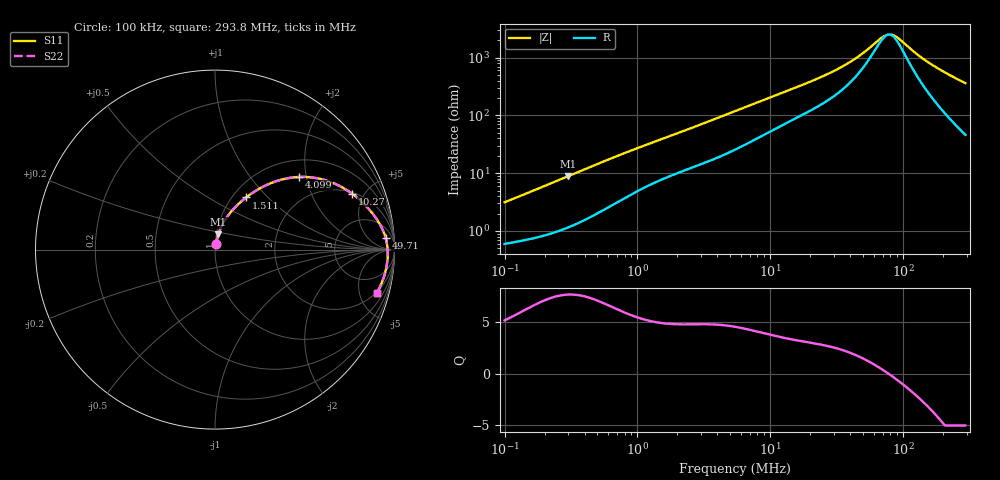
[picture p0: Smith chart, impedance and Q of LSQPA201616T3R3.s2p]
! LSQPA201616T3R3  S-PARAMETER MODEL  ( General Type )
! Model Generated by TAIYO YUDEN Corporation (http://www.ty-top.com)
! Version 2.0
! TAIYO YUDEN Control No. 100810NF25SB-FKC
! Copyright(c) 2007 TAIYO YUDEN CO.,LTD. All Rights Reserved.
! Product Description (link to TY-COMPAS)
! https://ds.yuden.co.jp/TYCOMPAS/or/detail?pn=LSQPA201616T3R3M&u=M
! Products Name : Inductors
! Characteristics :
!  Inductance : 3.3 uH , SRF(min) : 55 MHz , DC Resistance(max) : 0.351 Ohm
!  Rated Current : Saturation :600 mA , Temp Rise : 610 mA (40 degC)
!  Case Size : 2.0 x 1.6 / 0.079 x 0.063 [mm/inch] , Thickness : 1.6 / 0.063 [mm/inch]
!  (Conditions: Temperature = 25 degC , DC Bias Current/Voltage = 0A / 0V)
! External Node Assignments :
!  1  o---GGG---o  2
! GND o---------o GND
! Frequency Range : 0.1MHz  -  293.796821MHz  [ 402 STEP ]
# MHz S RI R 50
! Freq[MHz].  S11 Real  S11 Imag  S21 Real  S21 Imag  S12 Real  S12 Imag  S22 Real  S22 Imag
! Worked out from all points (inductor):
!   401 points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, 100 kHz to 293.8 MHz, reference 50 ohm
!   read as one part in series: L = 4.83 uH near 104.1 kHz
!   highest Q = 7.67 at 299.8 kHz (marker M1), where L = 4.67 uH
!   self-resonance near 77.77 MHz
!   S11 on the Smith chart (normalised r, x): 100 kHz: 1.01, +0.06; 1.511 MHz: 1.15, +0.76; 4.099 MHz: 1.38, +1.80; 10.27 MHz: 2.09, +4.07; 49.71 MHz: 14, +20; 293.8 MHz: 1.92, -7.17
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0.1  0.00687 0.0305  0.9931 -0.0305  0.9931 -0.0305  0.00687 0.0305
0.299817  0.0187 0.0853  0.9813 -0.0853  0.9813 -0.0853  0.0187 0.0853
0.380976  0.026 0.1062  0.974 -0.1062  0.974 -0.1062  0.026 0.1062
0.766217  0.0725 0.1894  0.9275 -0.1894  0.9275 -0.1894  0.0725 0.1894
1.451429  0.166 0.2845  0.834 -0.2845  0.834 -0.2845  0.166 0.2845
1.510553  0.1738 0.2907  0.8262 -0.2907  0.8262 -0.2907  0.1738 0.2907
2.43904  0.2903 0.3614  0.7097 -0.3614  0.7097 -0.3614  0.2903 0.3614
4.09866  0.4664 0.4046  0.5336 -0.4046  0.5336 -0.4046  0.4664 0.4046
5.420303  0.5702 0.3973  0.4298 -0.3973  0.4298 -0.3973  0.5702 0.3973
10.26756  0.7631 0.3121  0.2369 -0.3121  0.2369 -0.3121  0.7631 0.3121
20.65007  0.8821 0.1958  0.1179 -0.1958  0.1179 -0.1958  0.8821 0.1958
34.01531  0.9303 0.119  0.0697 -0.119  0.0697 -0.119  0.9303 0.119
49.70575  0.9511 0.0635  0.0489 -0.0635  0.0489 -0.0635  0.9511 0.0635
68.4114  0.9599 0.0182  0.0401 -0.0182  0.0401 -0.0182  0.9599 0.0182
74.09842  0.9611 0.00687  0.0389 -0.00687  0.0389 -0.00687  0.9611 0.00687
78.67184  0.9618 -0.00165  0.0382 0.00165  0.0382 0.00165  0.9618 -0.00165
83.52754  0.9622 -0.0102  0.0378 0.0102  0.0378 0.0102  0.9622 -0.0102
90.47116  0.9624 -0.0218  0.0376 0.0218  0.0376 0.0218  0.9624 -0.0218
127.0288  0.9591 -0.0734  0.0409 0.0734  0.0409 0.0734  0.9591 -0.0734
164.6697  0.9509 -0.1176  0.0491 0.1176  0.0491 0.1176  0.9509 -0.1176
222.1598  0.9326 -0.1762  0.0674 0.1762  0.0674 0.1762  0.9326 -0.1762
293.7968  0.9027 -0.2392  0.0973 0.2392  0.0973 0.2392  0.9027 -0.2392
